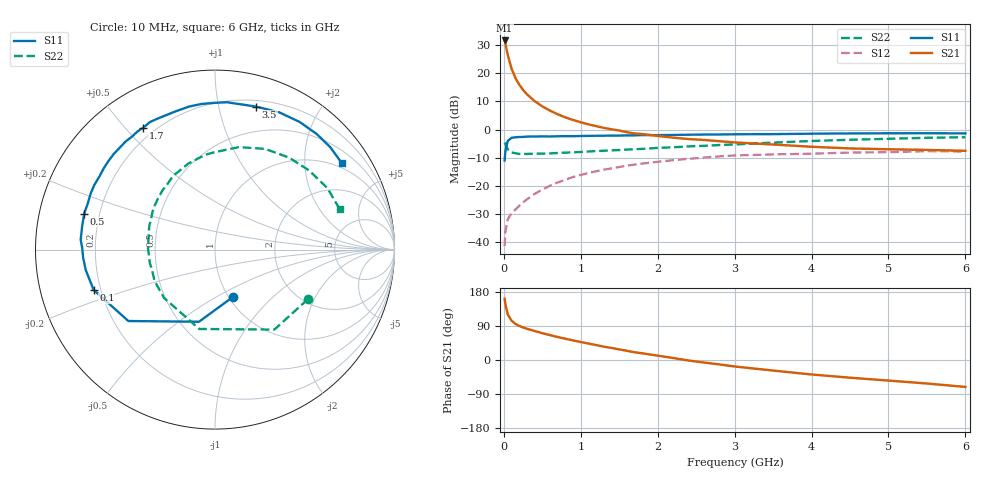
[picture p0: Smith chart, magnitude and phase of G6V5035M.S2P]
! SIEMENS Small Signal Semiconductors
! BFG193
! Si NPN RF Bipolar Junction Transistor in SOT223
! VCE = 0.5 V  IC = 35 mA
! Common Emitter S-Parameters:  August  1996
# GHz  S  MA  R  50
!  f  S11  S21  S12  S22
! GHz  MAG  ANG  MAG  ANG  MAG  ANG  MAG  ANG
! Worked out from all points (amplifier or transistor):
!   36 points, 10 MHz to 6 GHz, reference 50 ohm
!   highest |S21| = 31.6 dB at 10 MHz (marker M1)
!   |S21| within 3 dB of that: start of sweep to 34.36 MHz
!   unconditionally stable (mu >= 1): 209 MHz to end of sweep
!   at 250 MHz: K = 1.06, MAG = 18.5 dB, |S12| = -25.9 dB
!   at 1.4 GHz: K = 1.19, MAG = 4.3 dB, |S12| = -13.8 dB
!   at 6 GHz: K = 1.07, MAG = -1.5 dB, |S12| = -7.8 dB
!   S11 on the Smith chart (normalised r, x): 10 MHz: 1.04, -0.60; 100 MHz: 0.17, -0.16; 500 MHz: 0.14, +0.13; 1.7 GHz: 0.16, +0.56; 3.5 GHz: 0.25, +1.30; 6 GHz: 0.85, +3.04
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0.01  0.2828 -69.8  38.17 161.8  0.0085 72.8  0.5865 -28.2
0.02  0.4116 -102.5  33.59 147.4  0.0153 62.3  0.5549 -53.4
0.05  0.6257 -140.5  21.32 120.5  0.0254 46.0  0.4508 -101.2
0.1  0.7127 -161.7  12.11 103.8  0.0327 43.9  0.3913 -136.6
0.15  0.7292 -171.1  8.258 95.3  0.038 47.1  0.3794 -152.6
0.2  0.7362 -176.5  6.288 90.0  0.044 51.2  0.3692 -161.5
0.25  0.74 179.2  5.05 85.9  0.0508 53.1  0.3707 -168.6
0.3  0.7504 175.8  4.237 82.4  0.0578 55.2  0.3688 -172.8
0.4  0.7516 170.0  3.2 76.6  0.072 57.1  0.3729 179.2
0.5  0.7559 164.6  2.578 70.8  0.0859 56.7  0.3742 173.2
0.6  0.7539 160.3  2.166 65.7  0.1006 56.2  0.3774 168.5
0.7  0.7598 155.8  1.869 60.6  0.1149 54.9  0.3833 164.2
0.9  0.7618 147.8  1.48 51.7  0.1434 51.1  0.3936 155.5
1.1  0.7719 140.2  1.235 43.4  0.1689 47.0  0.4075 148.5
1.3  0.7771 133.1  1.069 35.1  0.194 42.3  0.4204 141.1
1.7  0.7881 120.4  0.852 20.4  0.239 32.4  0.4473 128.0
2.2  0.8012 105.7  0.718 5.3  0.2858 19.2  0.4837 113.3
2.8  0.8178 90.0  0.621 -11.6  0.3341 4.1  0.5309 96.0
3.5  0.829 74.0  0.542 -27.9  0.3621 -13.9  0.5861 76.9
4.5  0.8533 56.5  0.462 -46.7  0.3904 -32.5  0.6582 51.1
5.5  0.8591 41.6  0.435 -62.0  0.4128 -53.7  0.714 28.6
6  0.8552 34.2  0.419 -71.1  0.4076 -65.7  0.7306 17.9
